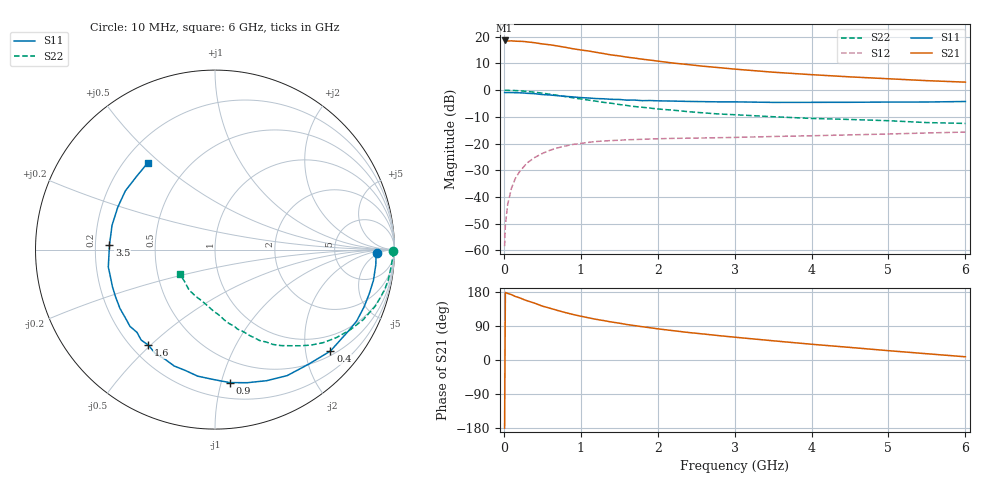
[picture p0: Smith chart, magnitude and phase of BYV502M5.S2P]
! SIEMENS Small Signal Semiconductors
! BFY420
! Si NPN RF SIEGET Grounded Emitter Transistor in MICRO-X
! VCE = 0.5 V  IC = 2.5 mA
! Common Emitter S-Parameters:  October  1996
# GHz  S  MA  R  50
!  f  S11  S21  S12  S22
! GHz  MAG  ANG  MAG  ANG  MAG  ANG  MAG  ANG
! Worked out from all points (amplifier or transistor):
!   36 points, 10 MHz to 6 GHz, reference 50 ohm
!   highest |S21| = 18.6 dB at 10 MHz (marker M1)
!   |S21| within 3 dB of that: start of sweep to 880.4 MHz
!   unconditionally stable (mu >= 1): 3.651 GHz to end of sweep
!   at 250 MHz: K = 0.07, MSG = 23.6 dB, |S12| = -29.0 dB
!   at 1.4 GHz: K = 0.38, MSG = 16.0 dB, |S12| = -18.9 dB
!   at 6 GHz: K = 1.27, MAG = 6.2 dB, |S12| = -15.7 dB
!   S11 on the Smith chart (normalised r, x): 10 MHz: 19, -4; 400 MHz: 0.60, -2.53; 900 MHz: 0.32, -1.06; 1.6 GHz: 0.27, -0.49; 3.5 GHz: 0.26, +0.02; 6 GHz: 0.29, +0.46
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0.01  0.9027 -1.2  8.486 -179.7  0.0012 98.3  0.9916 -0.6
0.02  0.8977 -2.4  8.439 178.2  0.003 82.3  0.9944 -1.3
0.05  0.8999 -5.3  8.305 175.6  0.0073 85.6  0.9898 -3.3
0.1  0.8994 -10.9  8.339 172.5  0.0147 84.9  0.9842 -6.6
0.15  0.894 -16.0  8.229 167.6  0.0223 80.0  0.9794 -9.9
0.25  0.884 -26.7  8.14 160.3  0.0355 73.7  0.9584 -16.3
0.3  0.8706 -31.5  7.997 156.5  0.043 72.1  0.9472 -19.4
0.4  0.8562 -41.3  7.691 150.0  0.0547 65.6  0.9135 -25.3
0.5  0.8241 -50.9  7.315 142.3  0.0651 60.3  0.8758 -30.7
0.6  0.8091 -60.2  7.037 136.6  0.0749 55.2  0.8358 -35.9
0.7  0.785 -68.5  6.688 130.7  0.0831 51.1  0.7961 -40.6
0.9  0.7455 -83.7  5.937 120.1  0.0962 43.3  0.7175 -48.3
1.1  0.7117 -97.8  5.389 111.4  0.1051 37.4  0.6499 -55.4
1.4  0.6712 -114.6  4.54 100.3  0.1136 30.0  0.5659 -63.7
1.6  0.6485 -124.9  4.134 93.6  0.1175 26.3  0.5147 -68.2
2  0.6294 -141.7  3.487 82.3  0.1228 21.0  0.4431 -75.6
2.2  0.6227 -148.3  3.204 77.4  0.1248 18.7  0.4206 -79.0
2.8  0.6019 -165.7  2.629 64.2  0.1287 14.4  0.3568 -88.1
3.5  0.5885 177.4  2.162 50.7  0.1354 11.2  0.3175 -97.1
4.5  0.5909 156.5  1.767 33.2  0.1451 6.7  0.2819 -112.3
5.5  0.5981 136.4  1.501 16.5  0.1575 2.9  0.2465 -133.1
6  0.6116 127.7  1.408 8.5  0.1639 0.9  0.2377 -145.3
